(* Logix 5000 AddOnInstructionDefinition export SPEL_PointCoordGet; software revision 30.01 *)

ADD_ON_INSTRUCTION SPEL_ExecCmd   (* revision 1.0 *)
// Executes a command in the robot controller.  Normally this is called by higher level AOIs.
VAR_INPUT
   Start : BOOL; {required}
   MaxTime : DINT := 3000; {required}
END_VAR
VAR_OUTPUT
   InCycle : BOOL; {access Read Only, visible}
   Done : BOOL; {access Read Only, visible}
   Error : BOOL; {access Read Only, visible}
END_VAR
VAR_IN_OUT
   ExtInputs : AB:ETHERNET_MODULE_INT_128Bytes:I:0; {required}
        .DATA[0].0   // ExtCmdGet
        .DATA[0].1   // ExtRespSet
        .DATA[0].2   // ExtCmdResult
        .DATA[0].3   // ExtError
   ExtOutputs : AB:ETHERNET_MODULE_INT_128Bytes:O:0; {required}
        .DATA[0].0   // ExtCmdSet
        .DATA[0].1   // ExtRespGet
        .DATA[0].2   // ExtCmdReset
END_VAR
VAR_INPUT
   Cmd : INT; {required}
   CmdParam1 : INT; {required}
   CmdParam2 : INT; {required}
   CmdParam3 : INT; {required}
   CmdParam4 : INT; {required}
   CmdParam5 : INT; {required}
   CmdParam6 : INT; {required}
   CmdParam7 : INT; {required}
END_VAR
VAR_OUTPUT
   CmdEcho : INT; {access Read Only, visible}
   Resp1 : INT; {access Read Only, visible}
   Resp2 : INT; {access Read Only, visible}
   Resp3 : INT; {access Read Only, visible}
   Resp4 : INT; {access Read Only, visible}
   Resp5 : INT; {access Read Only, visible}
   Resp6 : INT; {access Read Only, visible}
   Resp7 : INT; {access Read Only, visible}
   ErrCode1 : INT; {access Read Only, visible}
   ErrCode2 : INT; {access Read Only, visible}
END_VAR
VAR
   ExtReset : BOOL; {access None}
   ExtError : BOOL; {access None}
   ExtCmdSet : BOOL; {access None}   // Cmd Ready
   ExtCmdGet : BOOL; {access None}   // Cmd Received
   CmdXferDone : BOOL; {access None}
   ExtRespSet : BOOL; {access None}   // Resp Ready
   RespXferDone : BOOL; {access None}
   ExtCmdResult : BOOL; {access None}   // Normal or Error?
   TmrCmdDataRdy : TIMER := (PRE := 5); {access None}
   OneShotDoneOff : BOOL; {access None}
   OneShotStart : BOOL; {access None}
   StartInit : BOOL; {access None}
   OneShotStartError : BOOL; {access None}
   TmrCycle : TIMER := (PRE := 5000); {access None}
   OneshotTmrPreset : BOOL; {access None}
   TmrCmdSet : TIMER := (PRE := 20); {access None}
   OnShotCmdDataXfer : BOOL; {access None}
   OneShotRespDataXfer : BOOL; {access None}
   OneShotDataRdy : BOOL; {access None}
   OtherCmdInCycle : BOOL; {access None}
   s : BOOL; {access None}
   OneShotUnsetCmdIncycle : BOOL; {access None}
   OneShotSetCmdIncycle : BOOL; {access None}
   OneShotSetOtherCmdInCycleError : BOOL; {access None}
   OneShotSetBit : BOOL; {access None}
   MaxTimeError : BOOL; {access None}
END_VAR

ROUTINE Logic   (* ladder *)
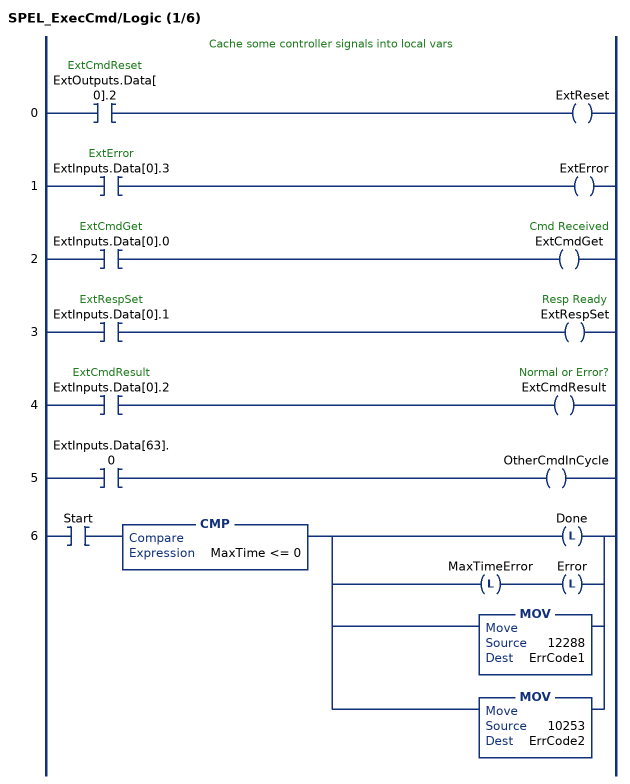
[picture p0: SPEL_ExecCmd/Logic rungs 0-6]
   // Cache some controller signals into local vars
   0: XIC(ExtOutputs.Data[0].2)OTE(ExtReset);
   1: XIC(ExtInputs.Data[0].3)OTE(ExtError);
   2: XIC(ExtInputs.Data[0].0)OTE(ExtCmdGet);
   3: XIC(ExtInputs.Data[0].1)OTE(ExtRespSet);
   4: XIC(ExtInputs.Data[0].2)OTE(ExtCmdResult);
   5: XIC(ExtInputs.Data[63].0)OTE(OtherCmdInCycle);
   6: XIC(Start)CMP(MaxTime <= 0)[OTL(Done) ,OTL(MaxTimeError) OTL(Error) ,MOV(12288,ErrCode1) ,MOV(10253,ErrCode2) ];
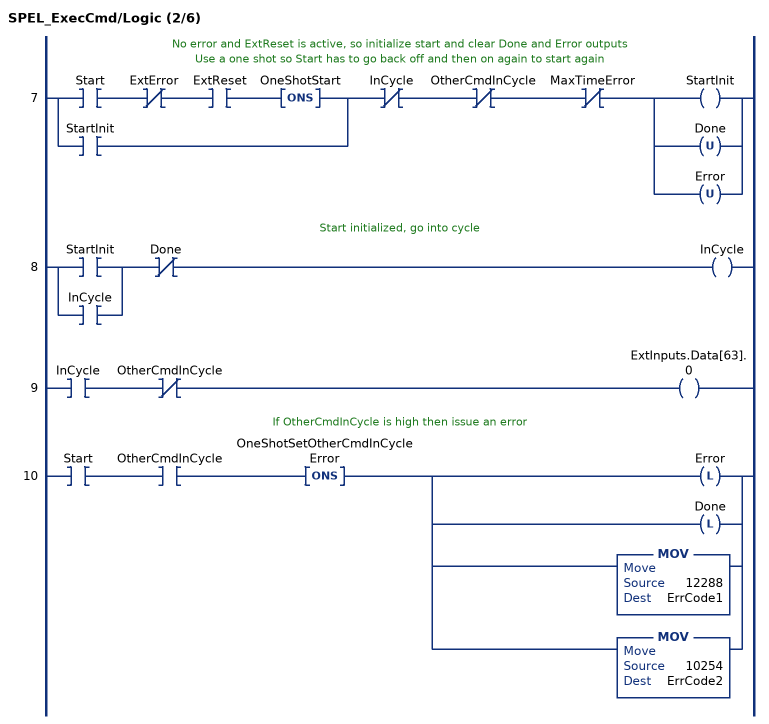
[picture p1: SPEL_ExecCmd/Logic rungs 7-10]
   // No error and ExtReset is active, so initialize start and clear Done and Error outputs
   // Use a one shot so Start has to go back off and then on again to start again
   7: [XIC(Start) XIO(ExtError) XIC(ExtReset) ONS(OneShotStart) ,XIC(StartInit) ]XIO(InCycle)XIO(OtherCmdInCycle)XIO(MaxTimeError)[OTE(StartInit) ,OTU(Done) ,OTU(Error) ];
   // Start initialized, go into cycle
   8: [XIC(StartInit) ,XIC(InCycle) ]XIO(Done)OTE(InCycle);
   9: XIC(InCycle)XIO(OtherCmdInCycle)OTE(ExtInputs.Data[63].0);
   // If OtherCmdInCycle is high then issue an error
   10: XIC(Start)XIC(OtherCmdInCycle)ONS(OneShotSetOtherCmdInCycleError)[OTL(Error) ,OTL(Done) ,MOV(12288,ErrCode1) ,MOV(10254,ErrCode2) ];
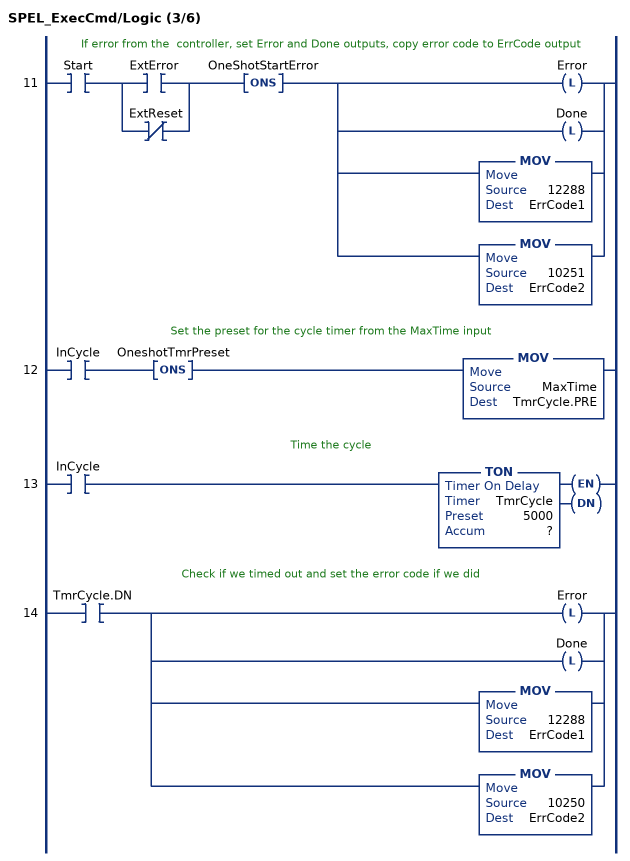
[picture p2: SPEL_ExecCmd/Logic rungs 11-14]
   // If error from the  controller, set Error and Done outputs, copy error code to ErrCode output
   11: XIC(Start)[XIC(ExtError) ,XIO(ExtReset) ]ONS(OneShotStartError)[OTL(Error) ,OTL(Done) ,MOV(12288,ErrCode1) ,MOV(10251,ErrCode2) ];
   // Set the preset for the cycle timer from the MaxTime input
   12: XIC(InCycle)ONS(OneshotTmrPreset)MOV(MaxTime,TmrCycle.PRE);
   // Time the cycle
   13: XIC(InCycle)TON(TmrCycle,?,?);
   // Check if we timed out and set the error code if we did
   14: XIC(TmrCycle.DN)[OTL(Error) ,OTL(Done) ,MOV(12288,ErrCode1) ,MOV(10250,ErrCode2) ];
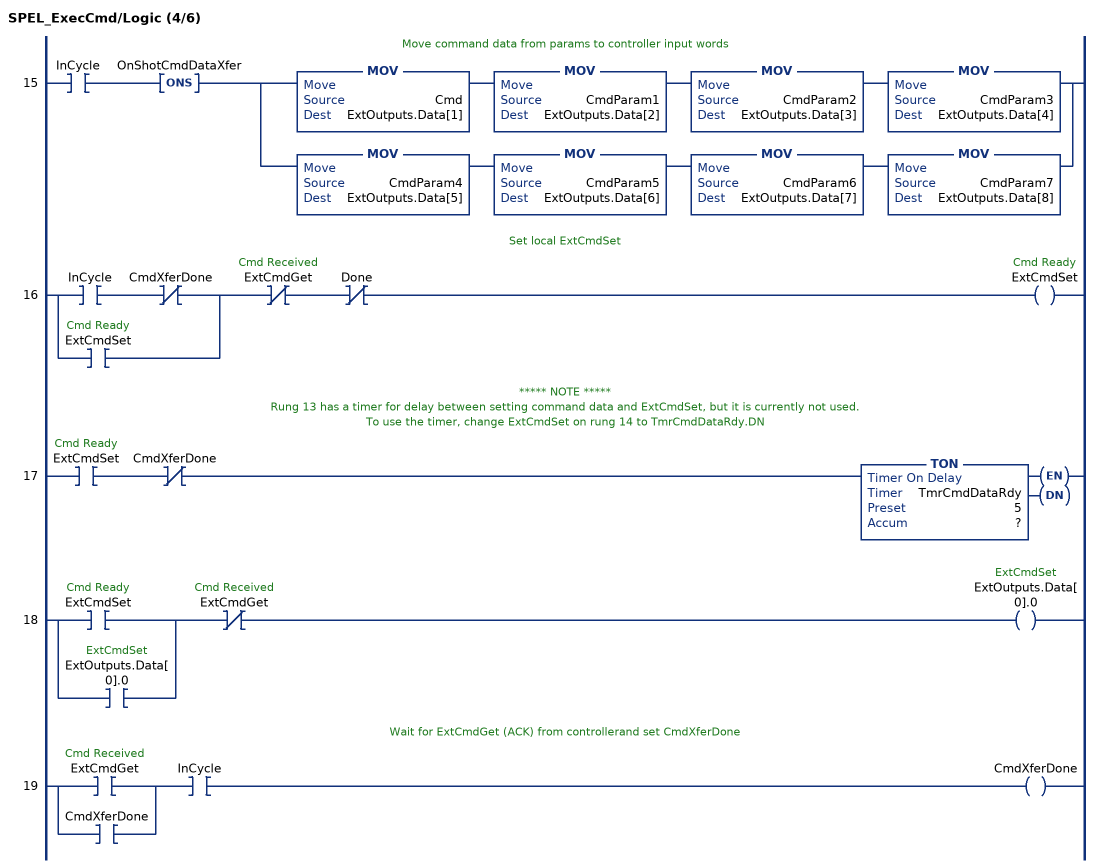
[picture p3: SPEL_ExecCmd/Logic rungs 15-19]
   // Move command data from params to controller input words
   15: XIC(InCycle)ONS(OnShotCmdDataXfer)[MOV(Cmd,ExtOutputs.Data[1]) MOV(CmdParam1,ExtOutputs.Data[2]) MOV(CmdParam2,ExtOutputs.Data[3]) MOV(CmdParam3,ExtOutputs.Data[4]) ,MOV(CmdParam4,ExtOutputs.Data[5]) MOV(CmdParam5,ExtOutputs.Data[6]) MOV(CmdParam6,ExtOutputs.Data[7]) MOV(CmdParam7,ExtOutputs.Data[8]) ];
   // Set local ExtCmdSet
   16: [XIC(InCycle) XIO(CmdXferDone) ,XIC(ExtCmdSet) ]XIO(ExtCmdGet)XIO(Done)OTE(ExtCmdSet);
   // ***** NOTE *****
   // Rung 13 has a timer for delay between setting command data and ExtCmdSet, but it is currently not used.
   // To use the timer, change ExtCmdSet on rung 14 to TmrCmdDataRdy.DN
   17: XIC(ExtCmdSet)XIO(CmdXferDone)TON(TmrCmdDataRdy,?,?);
   18: [XIC(ExtCmdSet) ,XIC(ExtOutputs.Data[0].0) ]XIO(ExtCmdGet)OTE(ExtOutputs.Data[0].0);
   // Wait for ExtCmdGet (ACK) from controllerand set CmdXferDone
   19: [XIC(ExtCmdGet) ,XIC(CmdXferDone) ]XIC(InCycle)OTE(CmdXferDone);
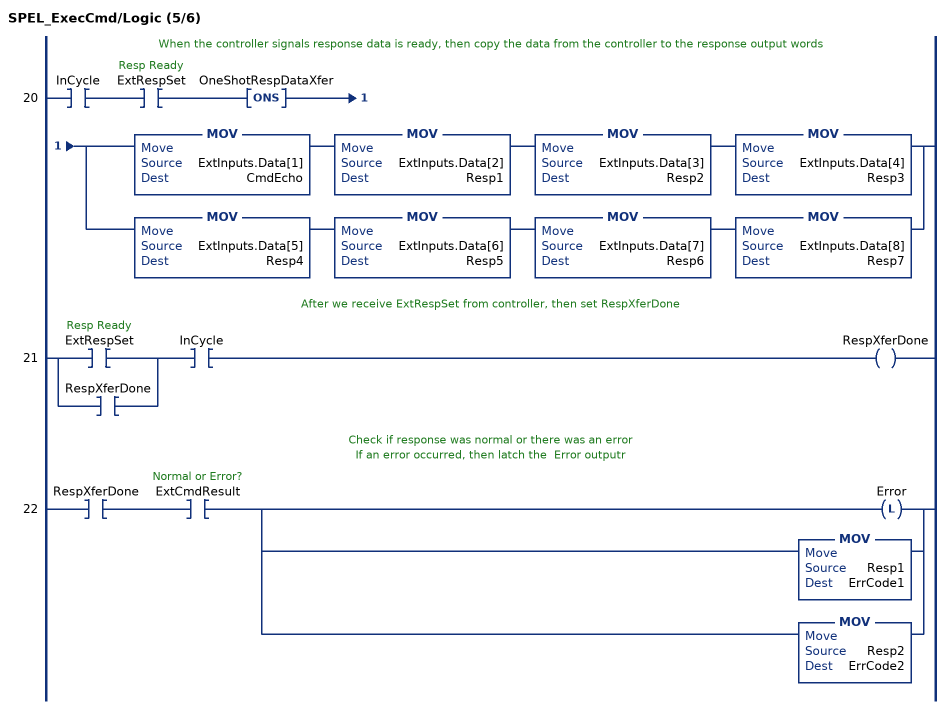
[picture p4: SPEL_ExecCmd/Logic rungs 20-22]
   // When the controller signals response data is ready, then copy the data from the controller to the response output words
   20: XIC(InCycle)XIC(ExtRespSet)ONS(OneShotRespDataXfer)[MOV(ExtInputs.Data[1],CmdEcho) MOV(ExtInputs.Data[2],Resp1) MOV(ExtInputs.Data[3],Resp2) MOV(ExtInputs.Data[4],Resp3) ,MOV(ExtInputs.Data[5],Resp4) MOV(ExtInputs.Data[6],Resp5) MOV(ExtInputs.Data[7],Resp6) MOV(ExtInputs.Data[8],Resp7) ];
   // After we receive ExtRespSet from controller, then set RespXferDone
   21: [XIC(ExtRespSet) ,XIC(RespXferDone) ]XIC(InCycle)OTE(RespXferDone);
   // Check if response was normal or there was an error
   // If an error occurred, then latch the  Error outputr
   22: XIC(RespXferDone)XIC(ExtCmdResult)[OTL(Error) ,MOV(Resp1,ErrCode1) ,MOV(Resp2,ErrCode2) ];
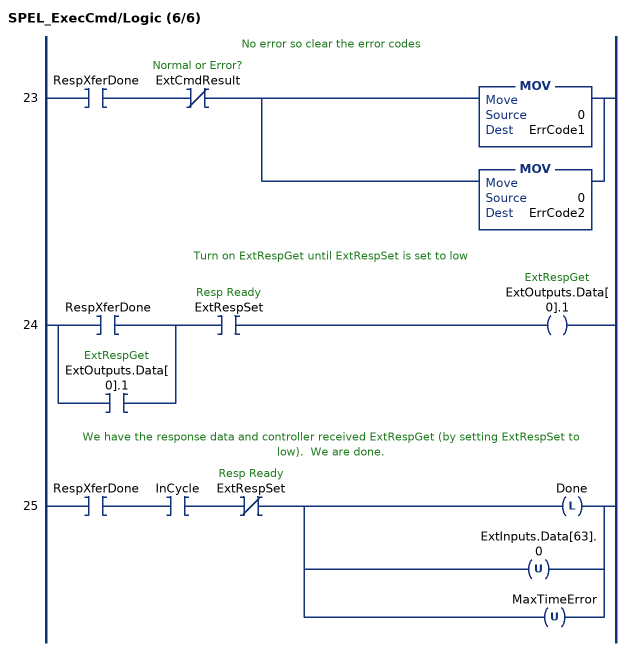
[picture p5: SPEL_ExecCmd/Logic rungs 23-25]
   // No error so clear the error codes
   23: XIC(RespXferDone)XIO(ExtCmdResult)[MOV(0,ErrCode1) ,MOV(0,ErrCode2) ];
   // Turn on ExtRespGet until ExtRespSet is set to low
   24: [XIC(RespXferDone) ,XIC(ExtOutputs.Data[0].1) ]XIC(ExtRespSet)OTE(ExtOutputs.Data[0].1);
   // We have the response data and controller received ExtRespGet (by setting ExtRespSet to low).  We are done.
   25: XIC(RespXferDone)XIC(InCycle)XIO(ExtRespSet)[OTL(Done) ,OTU(ExtInputs.Data[63].0) ,OTU(MaxTimeError) ];
END_ROUTINE
END_ADD_ON_INSTRUCTION

ADD_ON_INSTRUCTION SPEL_PointCoordGet   (* revision 1.2, vendor SEIKO EPSON CORP. *)
// Acquires the coordinate of the specified point.
VAR_OUTPUT
   InCycle : BOOL; {access Read Only, visible}
   Done : BOOL; {access Read Only, visible}
   Error : BOOL; {access Read Only, visible}
END_VAR
VAR_INPUT
   Start : BOOL; {access None, required}
   Point : INT; {access None, required}
   AxisNum : INT; {access None, required}
END_VAR
VAR_OUTPUT
   Value : REAL; {access Read Only, visible}
END_VAR
VAR_IN_OUT
   ExtInputs : AB:ETHERNET_MODULE_INT_128Bytes:I:0; {required}
   ExtOutputs : AB:ETHERNET_MODULE_INT_128Bytes:O:0; {required}
END_VAR
VAR_INPUT
   ErrCode1 : INT; {access None, visible}
   ErrCode2 : INT; {access None, visible}
END_VAR
VAR
   OneShotStart : BOOL; {access None}
   StartInit : BOOL; {access None}
   ExecGetPointCoord : SPEL_ExecCmd := (MaxTime := 3000); {access None}
   Coordinate_INTS : INT[2]; {access None}
   Coordinatex1000 : DINT; {access None}
END_VAR

ROUTINE Logic   (* ladder *)
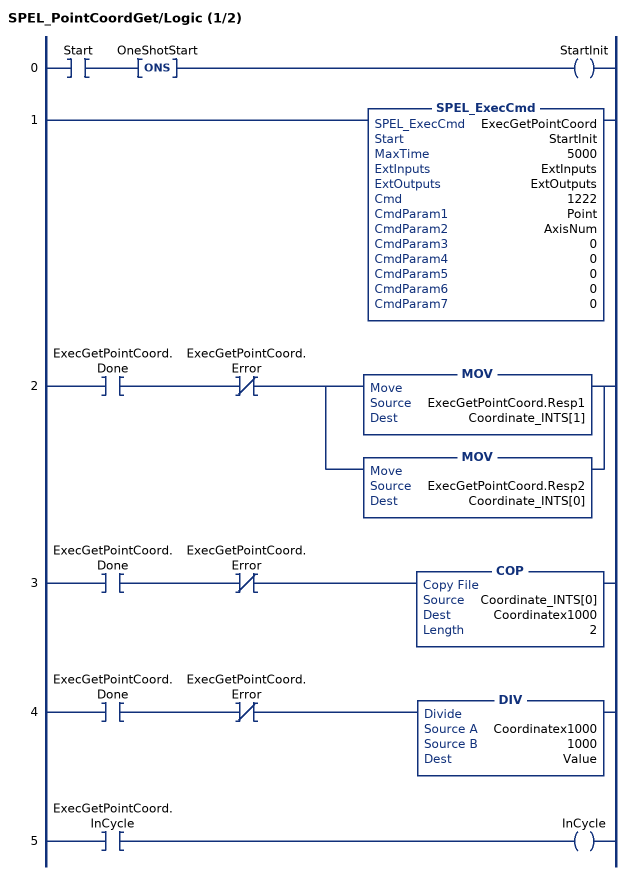
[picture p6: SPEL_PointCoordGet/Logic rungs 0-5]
   0: XIC(Start)ONS(OneShotStart)OTE(StartInit);
   1: SPEL_ExecCmd(ExecGetPointCoord,StartInit,5000,ExtInputs,ExtOutputs,1222,Point,AxisNum,0,0,0,0,0);
   2: XIC(ExecGetPointCoord.Done)XIO(ExecGetPointCoord.Error)[MOV(ExecGetPointCoord.Resp1,Coordinate_INTS[1]) ,MOV(ExecGetPointCoord.Resp2,Coordinate_INTS[0]) ];
   3: XIC(ExecGetPointCoord.Done)XIO(ExecGetPointCoord.Error)COP(Coordinate_INTS[0],Coordinatex1000,2);
   4: XIC(ExecGetPointCoord.Done)XIO(ExecGetPointCoord.Error)DIV(Coordinatex1000,1000,Value);
   5: XIC(ExecGetPointCoord.InCycle)OTE(InCycle);
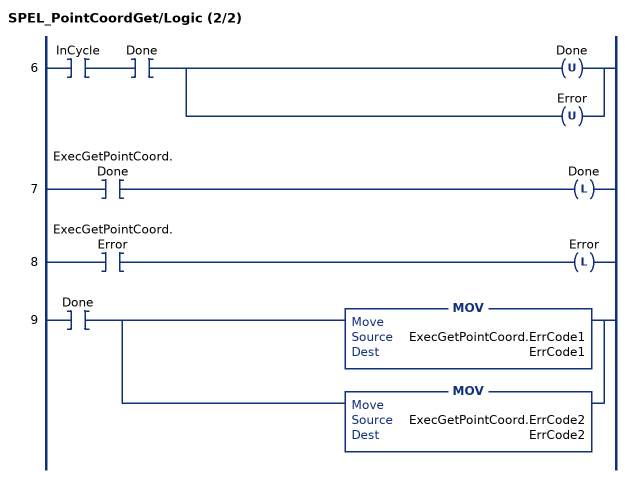
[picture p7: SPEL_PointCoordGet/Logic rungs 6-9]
   6: XIC(InCycle)XIC(Done)[OTU(Done) ,OTU(Error) ];
   7: XIC(ExecGetPointCoord.Done)OTL(Done);
   8: XIC(ExecGetPointCoord.Error)OTL(Error);
   9: XIC(Done)[MOV(ExecGetPointCoord.ErrCode1,ErrCode1) ,MOV(ExecGetPointCoord.ErrCode2,ErrCode2) ];
END_ROUTINE
END_ADD_ON_INSTRUCTION
